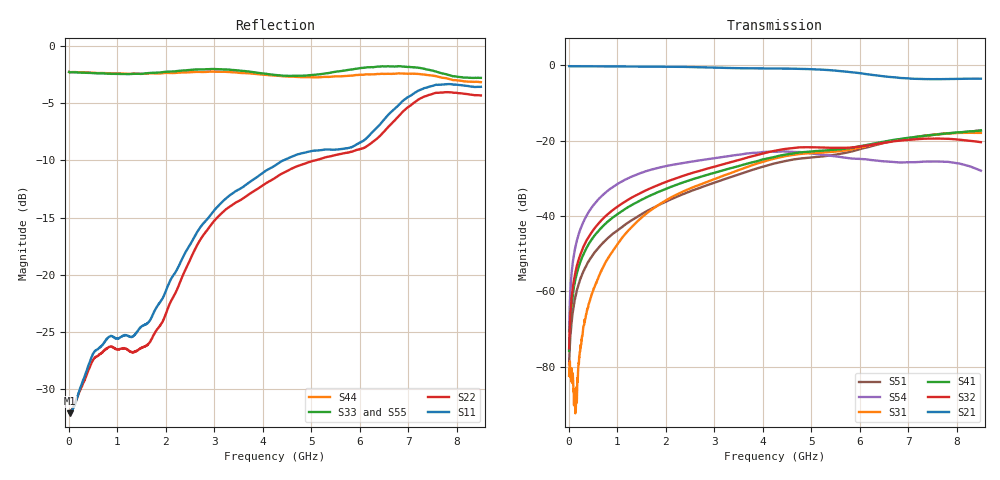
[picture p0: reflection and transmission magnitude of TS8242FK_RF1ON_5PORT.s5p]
! Created with skrf (http://scikit-rf.org).
# Hz S RI R 50.0
!freq ReS11 ImS11 ReS12 ImS12 ReS13 ImS13
! ReS14 ImS14 ReS15 ImS15
! ReS21 ImS21 ReS22 ImS22 ReS23 ImS23
! ReS24 ImS24 ReS25 ImS25
! ReS31 ImS31 ReS32 ImS32 ReS33 ImS33
! ReS34 ImS34 ReS35 ImS35
! ReS41 ImS41 ReS42 ImS42 ReS43 ImS43
! ReS44 ImS44 ReS45 ImS45
! ReS51 ImS51 ReS52 ImS52 ReS53 ImS53
! ReS54 ImS54 ReS55 ImS55
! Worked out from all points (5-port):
!   1601 points, 10 MHz to 8.5 GHz, reference 50 ohm
!   strongest paths, dB at 10 MHz, 2.132 GHz, 4.255 GHz, 6.378 GHz, 8.5 GHz:
!     S21: -0.2, -0.4, -0.9, -2.7, -3.6
!     S32: -75.2, -30.4, -22.7, -20.8, -20.4
!     S41: -75.8, -32.2, -24.3, -20.6, -17.3
!     S31: -82.5, -34.9, -24.7, -20.9, -18.0
!     S54: -70.6, -26.5, -23.0, -25.3, -28.0
!     S51: -79.3, -35.5, -26.0, -21.0, -17.3
!   lowest |S11| = -32.1 dB at 20.61 MHz (marker M1), VSWR 1.05, Z = 52.5 - j0.178 ohm
!   |S11| at or under -10 dB: start of sweep to 4.43 GHz
